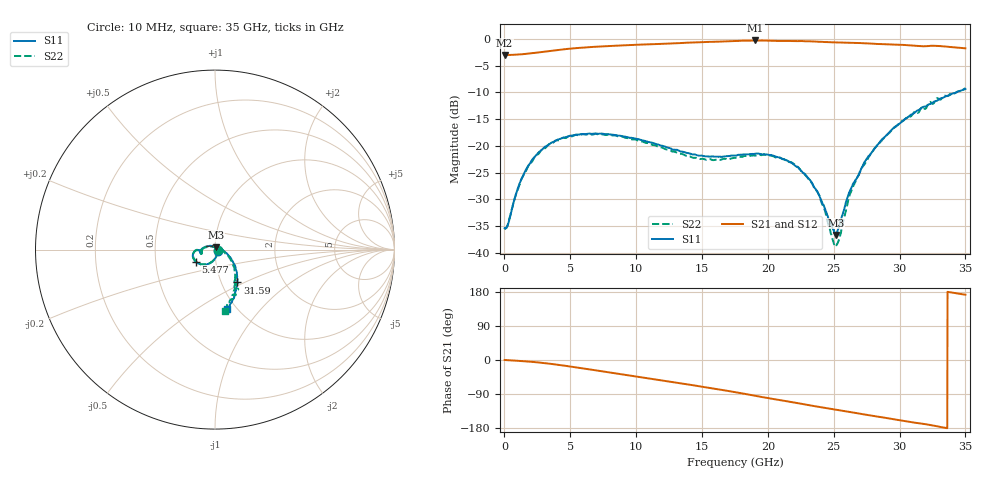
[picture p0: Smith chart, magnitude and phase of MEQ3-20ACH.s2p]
! MARKI MICROWAVE INC.
! Email:  support@markimicrowave.com  Phone:  408-778-4200
! Model Number:  MEQ3-20ACH  Date:  6/18
! Filename:		MEQ3-20ACH.S2P  Version: 1.0
! Description:  2-port S-parameter data for chip equalizer
! Features:		Low Insertion Loss, Excellent Return Loss
! Frequency Measured: 	10 MHz to 35 GHz
!S2P File: Measurements: S11, S21, S12, S22:
# Hz S  dB  R 50
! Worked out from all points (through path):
!   1601 points, 10 MHz to 35 GHz, reference 50 ohm
!   highest |S21| = -0.30 dB at 19.06 GHz (marker M1); lowest = -3.0 dB at 10 MHz (marker M2)
!   group delay of S21, straight-line fit = 15.6 ps
!   lowest |S11| = -36.7 dB at 25.16 GHz (marker M3), VSWR 1.03, Z = 50.6 + j1.34 ohm
!   |S11| at or under -10 dB: start of sweep to 34.33 GHz
!   |S22| runs from -38.8 to -9.2 dB; largest |S21 - S12| = 0.012
!   S11 on the Smith chart (normalised r, x): 10 MHz: 1.03, -0.01; 5.477 GHz: 0.80, -0.11; 31.59 GHz: 1.19, -0.46; 35 GHz: 0.90, -0.68
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1e7  -35.38 -18.7  -3.03 0.0  -2.99 -0.1  -35.53 -8.2
2.942938e8  -34.49 -36.2  -3.00 -0.6  -3.00 -0.7  -34.28 -35.3
1.278388e9  -26.31 -88.3  -2.89 -2.7  -2.88 -2.7  -26.25 -88.3
2.153138e9  -22.42 -106.9  -2.67 -5.1  -2.66 -5.1  -22.72 -107.4
3.8589e9  -19.08 -131.3  -2.14 -11.7  -2.14 -11.7  -19.04 -131.9
5.477188e9  -17.91 -148.0  -1.73 -19.7  -1.72 -19.7  -17.97 -148.1
5.848956e9  -17.81 -150.7  -1.65 -21.6  -1.65 -21.6  -17.89 -152.1
1.168791e10  -19.77 -178.3  -0.96 -52.4  -0.95 -52.4  -20.21 -179.7
1.483701e10  -21.84 -172.9  -0.63 -69.5  -0.63 -69.5  -22.46 -173.3
1.7505e10  -21.81 -165.8  -0.40 -84.8  -0.40 -84.9  -22.25 -163.4
1.905768e10  -21.49 -168.2  -0.30 -94.6  -0.30 -94.4  -21.82 -165.0
2.183501e10  -23.24 173.3  -0.41 -111.2  -0.43 -111.5  -23.16 176.7
2.334396e10  -26.93 156.0  -0.49 -120.5  -0.47 -120.3  -27.00 159.5
2.391254e10  -29.31 141.1  -0.55 -123.8  -0.51 -123.8  -29.33 150.2
2.515906e10  -36.68 65.0  -0.67 -131.0  -0.64 -131.4  -38.57 69.7
2.546522e10  -34.52 42.9  -0.68 -132.7  -0.69 -133.1  -36.95 38.7
2.62525e10  -28.37 3.4  -0.72 -137.3  -0.77 -137.4  -28.94 -3.9
2.69523e10  -25.21 -12.5  -0.79 -141.4  -0.81 -141.2  -25.04 -16.5
2.749902e10  -22.46 -20.7  -0.84 -144.7  -0.83 -144.4  -22.86 -23.7
2.918291e10  -17.59 -37.1  -1.03 -154.1  -1.01 -154.3  -17.67 -40.2
3.158848e10  -13.08 -55.7  -1.35 -167.5  -1.35 -167.4  -13.13 -59.5
3.5e10  -9.38 -78.4  -1.77 172.3  -1.67 172.9  -9.23 -80.6
